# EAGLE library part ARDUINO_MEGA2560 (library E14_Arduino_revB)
Device for representing an Arduino Mega 2560 board with a footprint in an EAGLE design. Created by Dave Young for Element14. More EAGLE documentation at: http://www.element14.com/community/community/knode/cadsoft_eagle
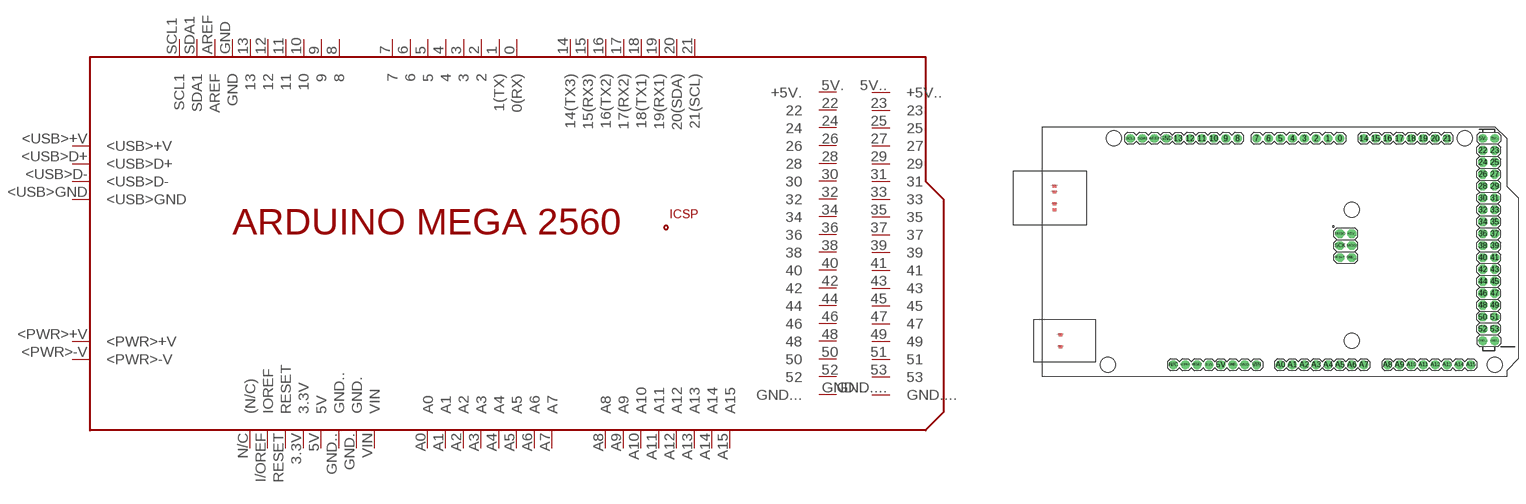
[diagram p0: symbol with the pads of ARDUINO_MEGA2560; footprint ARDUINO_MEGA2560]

Designator prefix PCB

## ARDUINO_MEGA2560  [ARDUINO_MEGA2560]
0  0(RX)
1  1(TX)
2  2
3  3
3.3V  3.3V
4  4
5  5
5V  5V
5V.  +5V.
5V..  +5V..
6  6
7  7
8  8
9  9
10  10
11  11
12  12
13  13
14  14(TX3)
15  15(RX3)
16  16(TX2)
17  17(RX2)
18  18(TX1)
19  19(RX1)
20  20(SDA)
21  21(SCL)
22  22
23  23
24  24
25  25
26  26
27  27
28  28
29  29
30  30
31  31
32  32
33  33
34  34
35  35
36  36
37  37
38  38
39  39
40  40
41  41
42  42
43  43
44  44
45  45
46  46
47  47
48  48
49  49
50  50
51  51
52  52
53  53
+5V_  +5V_
<PWR>+V  <PWR>+V  nc
<PWR>-V  <PWR>-V  nc
<USB>+V  <USB>+V  nc
<USB>D+  <USB>D+  nc
<USB>D-  <USB>D-  nc
<USB>GND  <USB>GND  nc
A0  A0
A1  A1
A2  A2
A3  A3
A4  A4
A5  A5
A6  A6
A7  A7
A8  A8
A9  A9
A10  A10
A11  A11
A12  A12
A13  A13
A14  A14
A15  A15
AREF  AREF
GND  GND
GND.  GND.
GND..  GND..
GND...  GND...
GND....  GND....
GND__  GND__
I/OREF  IOREF
MISO  MISO
MOSI  MOSI
N/C  (N/C)
RESET  RESET
RESET.  RESET.
SCK  SCK
SCL1  SCL1
SDA1  SDA1
VIN  VIN

## Footprint ARDUINO_MEGA2560 (pad centres in mm)
Footprint for representing an Arduino Mega board in an EAGLE schematic. Created by Dave Young for Element14. More EAGLE documentation at: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
drill 1.016 pad 1.88: 0 63.5,50.8; 1 60.96,50.8; 2 58.42,50.8; 3 55.88,50.8; 3.3V 35.56,2.54; 4 53.34,50.8; 5 50.8,50.8; 5V 38.1,2.54; 5V. 93.98,50.8; 5V.. 96.52,50.8; 6 48.26,50.8; 7 45.72,50.8; 8 41.656,50.8; 9 39.116,50.8; 10 36.576,50.8; 11 34.036,50.8; 12 31.496,50.8; 13 28.956,50.8; 14 68.58,50.8; 15 71.12,50.8; 16 73.66,50.8; 17 76.2,50.8; 18 78.74,50.8; 19 81.28,50.8; 20 83.82,50.8; 21 86.36,50.8; A0 50.8,2.54; A1 53.34,2.54; A2 55.88,2.54; A3 58.42,2.54; A4 60.96,2.54; A5 63.5,2.54; A6 66.04,2.54; A7 68.58,2.54; A8 73.66,2.54; A9 76.2,2.54; A10 78.74,2.54; A11 81.28,2.54; A12 83.82,2.54; A13 86.36,2.54; A14 88.9,2.54; A15 91.44,2.54; AREF 23.876,50.8; GND 26.416,50.8; GND. 43.18,2.54; GND.. 40.64,2.54; GND... 93.98,7.62; GND.... 96.52,7.62; I/OREF 30.48,2.54; N/C 27.94,2.54; RESET 33.02,2.54; SCL1 18.796,50.8; SDA1 21.336,50.8; VIN 45.72,2.54
drill 1.016 pad 1.88 octagon: 22 93.98,48.26; 23 96.52,48.26; 24 93.98,45.72; 25 96.52,45.72; 26 93.98,43.18; 27 96.52,43.18; 28 93.98,40.64; 29 96.52,40.64; 30 93.98,38.1; 31 96.52,38.1; 32 93.98,35.56; 33 96.52,35.56; 34 93.98,33.02; 35 96.52,33.02; 36 93.98,30.48; 37 96.52,30.48; 38 93.98,27.94; 39 96.52,27.94; 40 93.98,25.4; 41 96.52,25.4; 42 93.98,22.86; 43 96.52,22.86; 44 93.98,20.32; 45 96.52,20.32; 46 93.98,17.78; 47 96.52,17.78; 48 93.98,15.24; 49 96.52,15.24; 50 93.98,12.7; 51 96.52,12.7; 52 93.98,10.16; 53 96.52,10.16; +5V_ 66.04,30.48; GND__ 66.04,25.4; MISO 63.5,30.48; MOSI 66.04,27.94; RESET. 63.5,25.4; SCK 63.5,27.94
smd 1.016 x 0.508: <PWR>+V 3.81,8.89; <PWR>-V 3.81,6.35; <USB>+V 2.54,40.64; <USB>D+ 2.54,39.37; <USB>D- 2.54,36.83; <USB>GND 2.54,35.56
hole 3.2 at 15.24,50.8
hole 3.2 at 13.97,2.54
hole 3.2 at 66.04,35.56
hole 3.2 at 66.04,7.62
hole 3.2 at 90.17,50.8
hole 3.2 at 96.52,2.54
